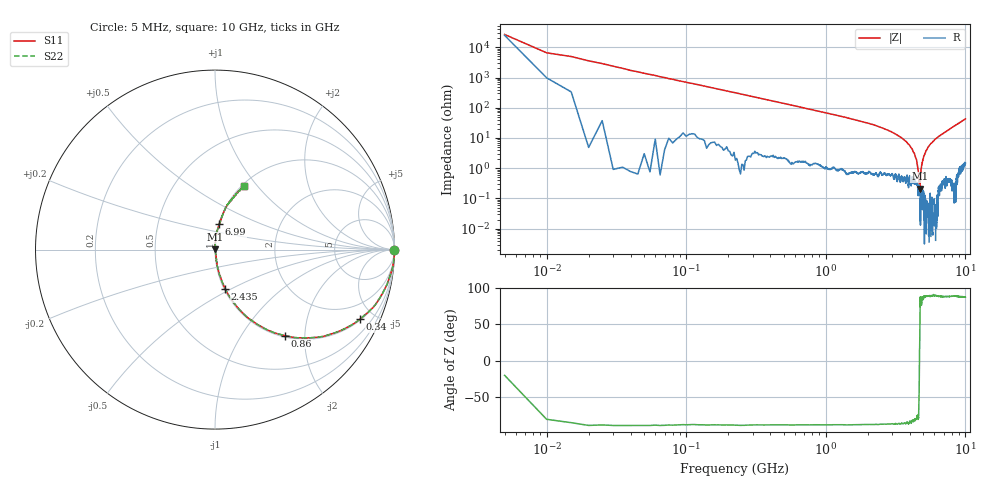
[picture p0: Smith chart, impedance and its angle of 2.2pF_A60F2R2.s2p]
! Amotech Co.,Ltd.
! http://www.amotech.co.kr/
! Part Number: A60F2R2
! These Parameters are Measured in Series Mode Connection
! Operation Temp=25[degC], DC Bias Voltage=0[V]
! Freq. Start=5[MHz] Stop=10[GHz], 2000[Steps]
! Date: Monday, July 20, 2020, 03:19:06
# GHZ S RI R 50.000000
!Freq.(Hz) S11(Real) S11(Imag) S21(Real) S21(Imag) S12(Real) S12(Imag) S22(Real) S22(Imag)
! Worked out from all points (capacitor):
!   2000 points, 5 MHz to 10 GHz, reference 50 ohm
!   read as one part in series: C = 2.28 pF near 55 MHz
!   lowest |Z| = 212 mohm at 4.715 GHz (marker M1)
!   series resonance near 4.69 GHz, so ESL is about 500 pH
!   S11 on the Smith chart (normalised r, x): 5 MHz: open; 340 MHz: 1.06, -4.12; 860 MHz: 1.03, -1.59; 2.435 GHz: 1.01, -0.47; 6.99 GHz: 1.01, +0.29; 10 GHz: 1.03, +0.86
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0.005  0.9965 -0.00131  0.00351 0.00131  0.00351 0.00131  0.9965 -0.00131
0.06  0.9921 -0.0845  0.00788 0.0845  0.00788 0.0845  0.9921 -0.0845
0.1  0.9778 -0.1393  0.0222 0.1393  0.0222 0.1393  0.9778 -0.1393
0.195  0.925 -0.2563  0.075 0.2563  0.075 0.2563  0.925 -0.2563
0.34  0.8059 -0.3888  0.1941 0.3888  0.1941 0.3888  0.8059 -0.3888
0.86  0.3905 -0.4792  0.6095 0.4792  0.6095 0.4792  0.3905 -0.4792
1.675  0.1353 -0.3332  0.8647 0.3332  0.8647 0.3332  0.1353 -0.3332
2.435  0.0575 -0.218  0.9425 0.218  0.9425 0.218  0.0575 -0.218
3.34  0.0193 -0.1126  0.9807 0.1126  0.9807 0.1126  0.0193 -0.1126
3.945  0.00724 -0.0595  0.9928 0.0595  0.9928 0.0595  0.00724 -0.0595
4.315  0.00496 -0.0299  0.995 0.0299  0.995 0.0299  0.00496 -0.0299
4.5  0.00338 -0.0149  0.9966 0.0149  0.9966 0.0149  0.00338 -0.0149
4.59  0.00131 -0.00845  0.9987 0.00845  0.9987 0.00845  0.00131 -0.00845
4.675  0.00226 -0.00118  0.9977 0.00118  0.9977 0.00118  0.00226 -0.00118
4.715  0.00155 0.00145  0.9985 -0.00145  0.9985 -0.00145  0.00155 0.00145
4.845  0.00239 0.011  0.9976 -0.011  0.9976 -0.011  0.00239 0.011
5.005  0.00224 0.0223  0.9978 -0.0223  0.9978 -0.0223  0.00224 0.0223
5.6  0.00506 0.062  0.9949 -0.062  0.9949 -0.062  0.00506 0.062
6.67  0.0185 0.1239  0.9815 -0.1239  0.9815 -0.1239  0.0185 0.1239
6.99  0.0237 0.1415  0.9763 -0.1415  0.9763 -0.1415  0.0237 0.1415
8.335  0.0613 0.2371  0.9387 -0.2371  0.9387 -0.2371  0.0613 0.2371
10  0.1643 0.3535  0.8357 -0.3535  0.8357 -0.3535  0.1643 0.3535
